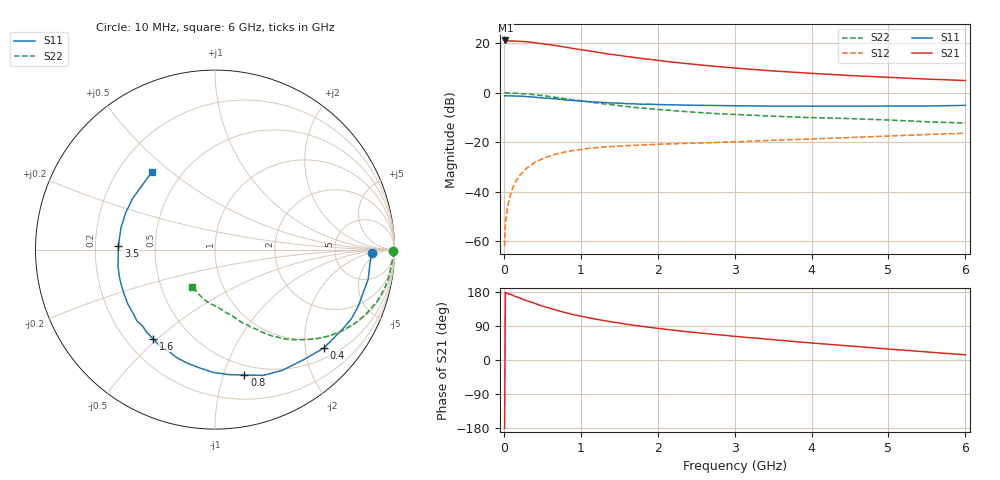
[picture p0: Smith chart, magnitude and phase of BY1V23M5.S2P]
! SIEMENS Small Signal Semiconductors
! BFY420
! Si NPN RF SIEGET Grounded Emitter Transistor in MICRO-X
! VCE = 1.25 V  IC = 3.5 mA
! Common Emitter S-Parameters:  October  1996
# GHz  S  MA  R  50
!  f  S11  S21  S12  S22
! GHz  MAG  ANG  MAG  ANG  MAG  ANG  MAG  ANG
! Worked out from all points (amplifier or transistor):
!   36 points, 10 MHz to 6 GHz, reference 50 ohm
!   highest |S21| = 21.1 dB at 20 MHz (marker M1)
!   |S21| within 3 dB of that: start of sweep to 855.7 MHz
!   unconditionally stable (mu >= 1): 3.423 GHz to end of sweep
!   at 250 MHz: K = 0.07, MSG = 26.3 dB, |S12| = -32.0 dB
!   at 1.4 GHz: K = 0.44, MSG = 18.6 dB, |S12| = -21.7 dB
!   at 6 GHz: K = 1.20, MAG = 7.9 dB, |S12| = -16.3 dB
!   S11 on the Smith chart (normalised r, x): 10 MHz: 14, -2; 400 MHz: 0.73, -2.41; 800 MHz: 0.41, -1.18; 1.6 GHz: 0.31, -0.48; 3.5 GHz: 0.30, +0.02; 6 GHz: 0.34, +0.43
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0.01  0.8737 -1.3  11.41 -179.9  0.0008 97.1  0.9942 -0.6
0.02  0.8708 -2.2  11.41 178.0  0.0023 95.6  0.9953 -1.2
0.05  0.8667 -5.6  11.18 175.5  0.0051 89.1  0.9902 -3.0
0.1  0.8692 -10.9  11.15 172.4  0.0106 86.1  0.9847 -6.0
0.15  0.8602 -16.2  11.07 167.4  0.0159 80.1  0.9801 -9.2
0.3  0.8378 -31.8  10.71 156.3  0.0304 73.0  0.9477 -17.8
0.4  0.8177 -42.1  10.29 149.7  0.039 67.0  0.9149 -23.2
0.5  0.7868 -51.3  9.751 142.2  0.0465 62.3  0.8785 -28.1
0.6  0.7704 -60.7  9.353 136.4  0.0535 58.1  0.8402 -32.6
0.7  0.751 -68.9  8.893 130.5  0.0591 54.1  0.8005 -36.8
0.8  0.718 -76.8  8.357 125.0  0.0642 49.9  0.76 -40.6
0.9  0.7002 -83.9  7.866 120.0  0.0685 46.8  0.7239 -43.7
1.1  0.6641 -97.7  7.078 111.6  0.0752 42.1  0.6579 -49.7
1.3  0.6386 -109.4  6.304 104.2  0.0804 37.8  0.6004 -54.3
1.6  0.6042 -124.9  5.404 94.2  0.0858 33.5  0.5294 -60.3
1.9  0.5889 -137.7  4.73 86.2  0.0897 30.4  0.4771 -65.2
2.2  0.5725 -148.2  4.151 78.8  0.0933 28.1  0.4377 -69.1
2.8  0.5531 -165.1  3.373 66.4  0.1002 25.5  0.3772 -76.2
3.5  0.5386 177.8  2.763 53.6  0.1097 23.6  0.3372 -83.5
4.5  0.5385 157.2  2.234 37.0  0.1248 20.2  0.3017 -95.3
5.5  0.5421 137.7  1.893 21.3  0.1438 16.0  0.2598 -111.6
6  0.5578 128.8  1.772 13.6  0.153 13.4  0.2452 -121.6
